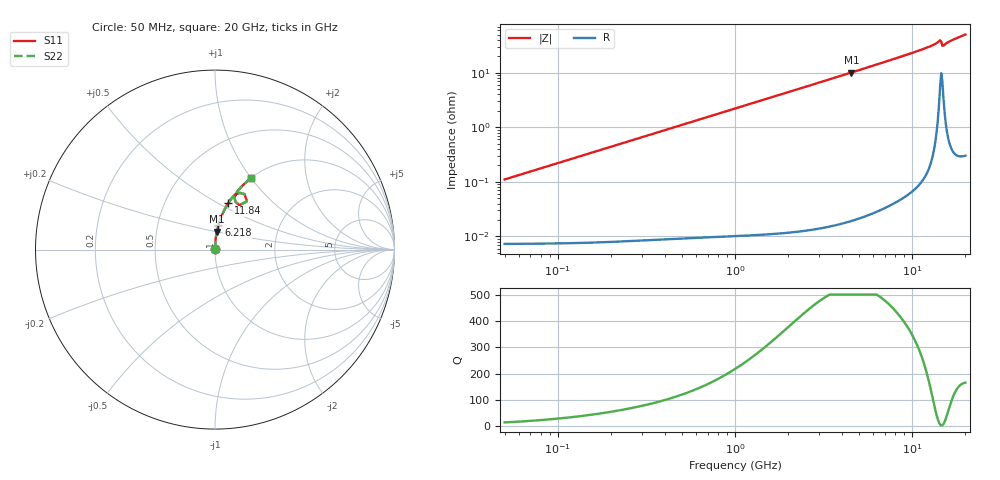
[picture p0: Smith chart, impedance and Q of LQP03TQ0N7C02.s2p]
!Murata Part Number: LQP03TQ0N7C02
!These Parameters are Measured in Series Mode Connection
!  o--[Z]--o
!Port1  Port2
!  o-------o
!Freq. Start=50[MHz] Stop=20[GHz], 401[Steps]
# Hz S RI R 50
!Freq.(Hz) S11(Real) S11(Imag) S21(Real) S21(Imag) S12(Real) S12(Imag) S22(Real) S22(Imag)
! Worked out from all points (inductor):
!   401 points, 50 MHz to 20 GHz, reference 50 ohm
!   read as one part in series: L = 352 pH near 51.52 MHz
!   highest Q = 526 at 4.54 GHz (marker M1), where L = 354 pH
!   S11 on the Smith chart (normalised r, x): 50 MHz: 1.00, +0.00; 6.218 GHz: 1.00, +0.28; 11.84 GHz: 1.00, +0.56; 20 GHz: 1.01, +1.00
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5e7  7.41e-05 0.00111  0.9999 -0.00111  0.9999 -0.00111  7.41e-05 0.00111
1.364002e8  8.52e-05 0.00301  0.9999 -0.00301  0.9999 -0.00301  8.52e-05 0.00301
3.721004e8  0.000155 0.00821  0.9998 -0.00821  0.9998 -0.00821  0.000155 0.00821
1e9  0.000587 0.022  0.9994 -0.022  0.9994 -0.022  0.000587 0.022
1.714689e9  0.00154 0.0378  0.9985 -0.0378  0.9985 -0.0378  0.00154 0.0378
2.728004e9  0.00375 0.06  0.9962 -0.06  0.9962 -0.06  0.00375 0.06
4.539627e9  0.0103 0.0998  0.9897 -0.0998  0.9897 -0.0998  0.0103 0.0998
6.217679e9  0.0193 0.1365  0.9807 -0.1365  0.9807 -0.1365  0.0193 0.1365
7.442007e9  0.0277 0.1631  0.9723 -0.1631  0.9723 -0.1631  0.0277 0.1631
9.600142e9  0.0468 0.2099  0.9532 -0.2099  0.9532 -0.2099  0.0468 0.2099
1.183995e10  0.0736 0.259  0.9264 -0.259  0.9264 -0.259  0.0736 0.259
1.314879e10  0.0962 0.2899  0.9038 -0.2899  0.9038 -0.2899  0.0962 0.2899
1.354865e10  0.1067 0.3005  0.8933 -0.3005  0.8933 -0.3005  0.1067 0.3005
1.396067e10  0.124 0.312  0.876 -0.312  0.876 -0.312  0.124 0.312
1.417136e10  0.1396 0.316  0.8604 -0.316  0.8604 -0.316  0.1396 0.316
1.438523e10  0.1643 0.3093  0.8357 -0.3093  0.8357 -0.3093  0.1643 0.3093
1.482269e10  0.1361 0.2473  0.8639 -0.2473  0.8639 -0.2473  0.1361 0.2473
1.504638e10  0.113 0.2677  0.887 -0.2677  0.887 -0.2677  0.113 0.2677
1.527346e10  0.1099 0.2862  0.8901 -0.2862  0.8901 -0.2862  0.1099 0.2862
1.597544e10  0.1207 0.3171  0.8793 -0.3171  0.8793 -0.3171  0.1207 0.3171
1.670968e10  0.135 0.3367  0.865 -0.3367  0.865 -0.3367  0.135 0.3367
2e10  0.203 0.3992  0.797 -0.3992  0.797 -0.3992  0.203 0.3992
